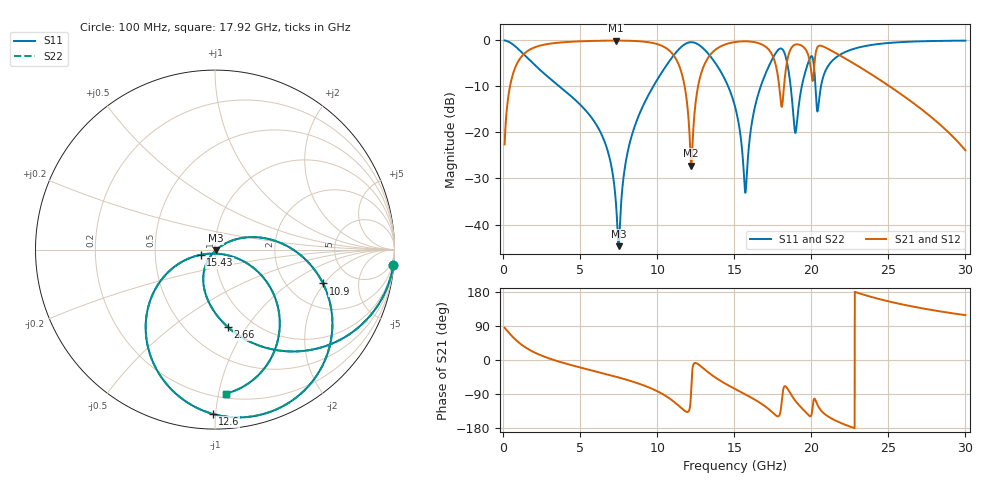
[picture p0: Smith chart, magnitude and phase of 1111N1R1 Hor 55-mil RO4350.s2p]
# GHz S MA R 50
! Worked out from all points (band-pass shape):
!   3201 points, 100 MHz to 30 GHz, reference 50 ohm
!   highest |S21| = -0.06 dB at 7.313 GHz (marker M1); lowest = -27.2 dB at 12.21 GHz (marker M2)
!   |S21| within 3 dB of the highest: 1.324 GHz to 11.02 GHz (9.698 GHz wide, 157 % of centre); 13.46 GHz to 17.45 GHz (3.984 GHz wide, 25.8 % of centre)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
!   lowest |S11| = -44.7 dB at 7.5 GHz (marker M3), VSWR 1.01, Z = 50.4 - j0.4 ohm
!   |S11| at or under -10 dB: 3.657 GHz to 9.745 GHz (6.089 GHz wide, 90.9 % of centre); 14.61 GHz to 16.72 GHz (2.111 GHz wide, 13.5 % of centre); 18.66 GHz to 19.38 GHz (722.4 MHz wide, 3.8 % of centre)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
!   |S22| runs from -44.7 to 0.0 dB; largest |S21 - S12| = 0
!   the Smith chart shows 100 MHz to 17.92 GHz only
!   S11 on the Smith chart (normalised r, x): 100 MHz: 1, -23; 2.66 GHz: 0.77, -0.82; 10.9 GHz: 3.10, -1.94; 12.6 GHz: 0.09, -0.98; 15.43 GHz: 0.85, -0.05; 17.92 GHz: 0.23, -1.05
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0.1  0.9972 -4.9  0.07411 85.1  0.07411 85.1  0.9972 -4.9
0.8475  0.845 -37.7  0.5338 52.3  0.5338 52.3  0.845 -37.7
2.660188  0.4364 -80.7  0.8974 9.0  0.8974 9.0  0.4364 -80.7
5.089563  0.1939 -109.6  0.977 -20.6  0.977 -20.6  0.1939 -109.6
7.313375  0.01808 -116.2  0.9935 -44.0  0.9935 -44.0  0.01808 -116.2
7.50025  0.005822 -43.0  0.9933 -46.1  0.9933 -46.1  0.005822 -43.0
8.275781  0.08337 29.6  0.9883 -55.3  0.9883 -55.3  0.08337 29.6
10.06978  0.3898 3.9  0.903 -83.7  0.903 -83.7  0.3898 3.9
10.90137  0.6304 -17.4  0.7423 -104.4  0.7423 -104.4  0.6304 -17.4
12.2095  0.955 -72.3  0.0437 -75.2  0.0437 -75.2  0.955 -72.3
12.60194  0.9153 -90.8  0.2836 -9.6  0.2836 -9.6  0.9153 -90.8
15.05  0.1915 -159.9  0.9585 -76.4  0.9585 -76.4  0.1915 -159.9
15.43309  0.08559 -160.1  0.9734 -84.6  0.9734 -84.6  0.08559 -160.1
15.75078  0.0236 -71.9  0.976 -91.4  0.976 -91.4  0.0236 -71.9
16.45156  0.2248 -24.7  0.9447 -107.4  0.9447 -107.4  0.2248 -24.7
17.91853  0.8049 -85.8  0.3164 -146.6  0.3164 -146.6  0.8049 -85.8
18.39506  0.6083 -132.9  0.5481 -72.1  0.5481 -72.1  0.6083 -132.9
18.97437  0.09886 -97.4  0.9007 -108.1  0.9007 -108.1  0.09886 -97.4
20.03956  0.6722 -96.8  0.3926 -139.2  0.3926 -139.2  0.6722 -96.8
20.44134  0.1818 -77.1  0.8597 -121.5  0.8597 -121.5  0.1818 -77.1
25.01978  0.9366 -116.6  0.322 154.7  0.322 154.7  0.9366 -116.6
30  0.9926 -153.5  0.06391 118.4  0.06391 118.4  0.9926 -153.5
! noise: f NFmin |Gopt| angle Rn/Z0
0.1  0.002818  0.9432  2.27  0.01109
3.417  0.01302  0.5845  24.67  0.005473
6.743  0.0246  0.5741  42.27  0.009207
10.06  0.05689  0.7098  59.19  0.02945
13.39  0.1207  0.8119  79.98  0.07915
16.7  0.1008  0.7325  94.86  0.03538
20.03  0.6118  0.9411  112.1  0.729
23.35  0.139  0.7481  123.2  0.02691
26.67  0.2443  0.8487  138.3  0.04552
30  0.6586  0.9428  155  0.1231
